PROGRAM MAIN
VAR
	master,slave:					axis_ref;
	camming_state: 					camming_state;
	
	camin:							mc_camin;(*用于电子凸轮耦合功能块*)
	camout:							mc_camout;(*用于电子凸轮表解耦功能块*)
	CamTableSelect_1:				MC_CamTableSelect;(*用于创建凸轮表*)
	cam_table1:						MC_CAM_REF;(*用于定义凸轮表*)
	table1: 						ARRAY[1..5] OF MC_MotionFunctionPoint; (*用于定义电子凸轮表中的关键点，此例子中包含五个关键点*)
	CamInOut,CamOutOut,selectOut:	ST_McOutputs;(*用于绑定相关功能块输出接口*)

	move_velo_master:				mc_movevelocity;
	move_abs_slave:					mc_moveabsolute;
	MoveMasterOut:					ST_McOutputs;		
	MoveSlaveOut:					ST_McOutputs;	

	ResetSlave,resetMaster:			mc_reset;	
	ResetMasterOut,ResetSlaveOut:	ST_McOutputs;
	
	master_actpos,slave_actpos:		LREAL;
END_VAR

(*用于更新轴状态*)
master();
slave();

power();
camming();
reset();
move_m_s();
table1_point();	

CASE camming_state OF
	state_init:(*程序初始化*)
		move_velo_master.Execute := FALSE;
		ResetMaster.Execute := FALSE;
		ResetSlave.Execute := FALSE;
		CamIn.Execute := FALSE;
		CamOut.Execute := FALSE;
		camming_state:=state_power;
	
	state_power:(*主从轴使能*)
		IF master.NcToPlc.StateDWord.0 AND master.NcToPlc.StateDWord.0 THEN
			camming_state := state_forward;
		ELSIF master.Status.Error OR slave.Status.Error THEN
			camming_state := state_error;
		END_IF	
	
	state_forward:(*主轴100正转，从轴回0*)
			move_velo_master.Execute:=TRUE;
			move_abs_slave. Execute:=TRUE;
			IF master.Status.Moving AND move_abs_slave.Done  THEN
				move_velo_master.Execute:=FALSE;
				move_abs_slave.Execute:=FALSE;
				camming_state:=state_pre_table1;
			END_IF
		IF master.Status.Error OR slave.Status.Error THEN
			camming_state := state_error;
		END_IF	
		
	state_pre_table1:(*table1初始化*)
		camtableselect_1.Execute:=TRUE;
		camin.CamTableID:=1;
		IF camtableselect_1.Done THEN
			camming_state:=state_camming1;
			camtableselect_1.Execute:=FALSE;
		END_IF
		IF master.Status.Error OR slave.Status.Error THEN
			camming_state := state_error;
		END_IF
	
	state_camming1:
		camin.Execute:=TRUE;
		IF camin.InSync THEN			
			camin.Execute:=FALSE;
			camming_state:=camming_status;		
		END_IF
		IF master.Status.Error OR slave.Status.Error THEN
			camming_state := state_error;
		END_IF
		
	camming_status:
		master_actpos:=master.NcToPlc.SetPos;
		slave_actpos:=slave.NcToPlc.SetPos;		
		IF master.Status.Error OR slave.Status.Error THEN
			camming_state := state_error;
		END_IF
		
	state_error:
		CamOut.Execute := Slave.Status.Coupled; (* 先解耦 *)		
		IF not Slave.Status.Coupled THEN
			IF Master.Status.Error OR Slave.Status.Error THEN
				camming_state := state_reset;	(* 轴报错需要reset*)
			ELSE
				camming_state  := state_init;(*若功能块报错，不需要reset*)
			END_IF
		END_IF
	
	state_reset:
		ResetMaster.Execute := TRUE;
		CamTableSelect_1.Execute:=FALSE;
			ResetSlave.Execute := TRUE;
			IF ResetMaster.Done AND ResetSlave.Done THEN
				camming_state := state_init;
			ELSIF ResetMaster.Error OR ResetSlave.Error THEN
				camming_state := state_init; 
			END_IF
	
END_CASE

ACTION camming:
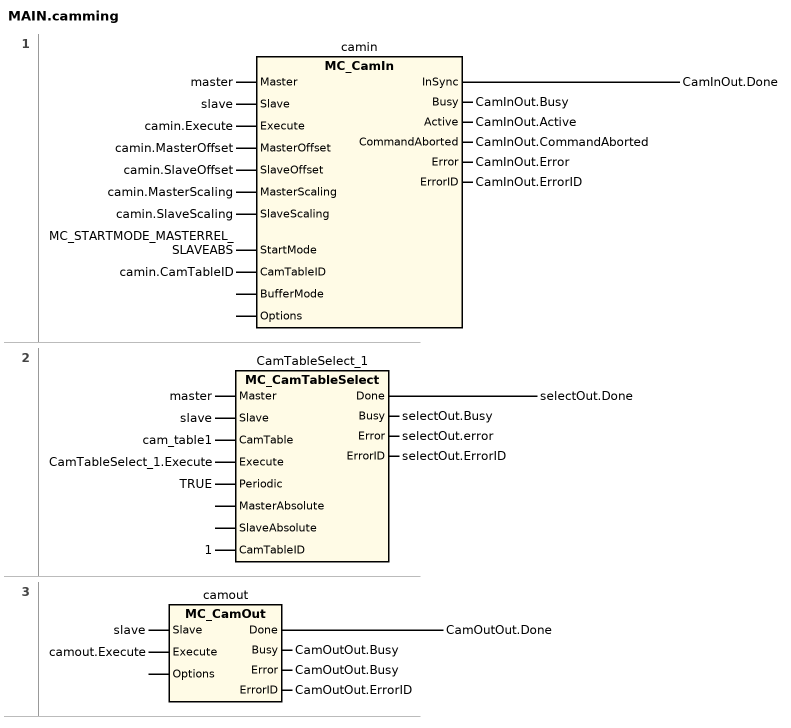
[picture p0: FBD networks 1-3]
// NETWORK 1
camin(
    Master := master,
    Slave := slave,
    Execute := camin.Execute,
    MasterOffset := camin.MasterOffset,
    SlaveOffset := camin.SlaveOffset,
    MasterScaling := camin.MasterScaling,
    SlaveScaling := camin.SlaveScaling,
    StartMode := MC_STARTMODE_MASTERREL_SLAVEABS,
    CamTableID := camin.CamTableID,
    Busy => CamInOut.Busy,
    Active => CamInOut.Active,
    CommandAborted => CamInOut.CommandAborted,
    Error => CamInOut.Error,
    ErrorID => CamInOut.ErrorID); // MC_CamIn
CamInOut.Done := camin.InSync;

// NETWORK 2
CamTableSelect_1(
    Master := master,
    Slave := slave,
    CamTable := cam_table1,
    Execute := CamTableSelect_1.Execute,
    Periodic := TRUE,
    CamTableID := 1,
    Busy => selectOut.Busy,
    Error => selectOut.error,
    ErrorID => selectOut.ErrorID); // MC_CamTableSelect
selectOut.Done := CamTableSelect_1.Done;

// NETWORK 3
camout(
    Slave := slave,
    Execute := camout.Execute,
    Busy => CamOutOut.Busy,
    Error => CamOutOut.Busy,
    ErrorID => CamOutOut.ErrorID); // MC_CamOut
CamOutOut.Done := camout.Done;
END_ACTION

ACTION move_m_s:
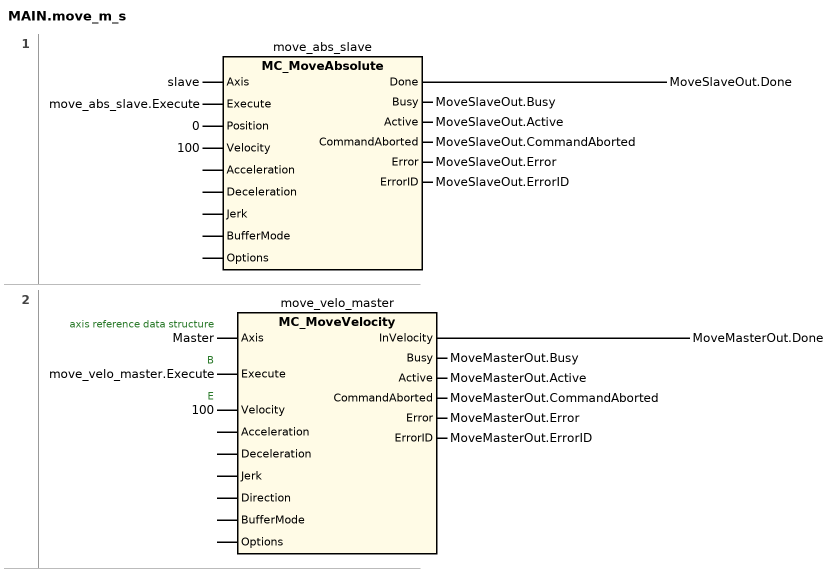
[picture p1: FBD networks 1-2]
// NETWORK 1
move_abs_slave(
    Axis := slave,
    Execute := move_abs_slave.Execute,
    Position := 0,
    Velocity := 100,
    Busy => MoveSlaveOut.Busy,
    Active => MoveSlaveOut.Active,
    CommandAborted => MoveSlaveOut.CommandAborted,
    Error => MoveSlaveOut.Error,
    ErrorID => MoveSlaveOut.ErrorID); // MC_MoveAbsolute
MoveSlaveOut.Done := move_abs_slave.Done;

// NETWORK 2
//   Master: axis reference data structure
//   move_velo_master.Execute: B
//   100: E
move_velo_master(
    Axis := Master,
    Execute := move_velo_master.Execute,
    Velocity := 100,
    Busy => MoveMasterOut.Busy,
    Active => MoveMasterOut.Active,
    CommandAborted => MoveMasterOut.CommandAborted,
    Error => MoveMasterOut.Error,
    ErrorID => MoveMasterOut.ErrorID); // MC_MoveVelocity
MoveMasterOut.Done := move_velo_master.InVelocity;
END_ACTION

ACTION power:
master.PlcToNc.ControlDWord:=7;
slave.PlcToNc.ControlDWord:=7;

master.PlcToNc.Override:=1000000;
slave.PlcToNc.Override:=1000000;
END_ACTION

ACTION reset:
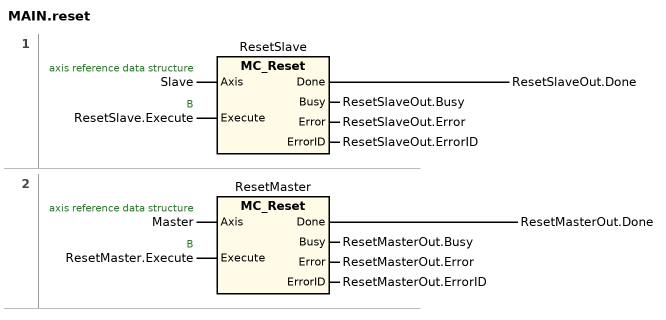
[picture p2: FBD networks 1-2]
// NETWORK 1
//   Slave: axis reference data structure
//   ResetSlave.Execute: B
ResetSlave(
    Axis := Slave,
    Execute := ResetSlave.Execute,
    Busy => ResetSlaveOut.Busy,
    Error => ResetSlaveOut.Error,
    ErrorID => ResetSlaveOut.ErrorID); // MC_Reset
ResetSlaveOut.Done := ResetSlave.Done;

// NETWORK 2
//   Master: axis reference data structure
//   ResetMaster.Execute: B
ResetMaster(
    Axis := Master,
    Execute := ResetMaster.Execute,
    Busy => ResetMasterOut.Busy,
    Error => ResetMasterOut.Error,
    ErrorID => ResetMasterOut.ErrorID); // MC_Reset
ResetMasterOut.Done := ResetMaster.Done;
END_ACTION

ACTION table1_point:
cam_table1.ArraySize:=SIZEOF(table1);
cam_table1.NoOfColumns:=1;
cam_table1.NoOfRows:=5;
cam_table1.pArray:=ADR(table1);
cam_table1.TableType:=MC_TABLETYPE_MOTIONFUNCTION;

		
table1[1].FunctionType:=MOTIONFUNCTYPE_POLYNOM5;
table1[1].MasterPos:=0;
table1[1].SlavePos:=0;
table1[1].PointIndex:=1;
table1[1].PointType:=MOTIONPOINTTYPE_MOTION;
		
table1[2].FunctionType:=MOTIONFUNCTYPE_POLYNOM5;
table1[2].MasterPos:=90;
table1[2].SlavePos:=100;
table1[2].PointIndex:=2;
table1[2].PointType:=MOTIONPOINTTYPE_MOTION;
		
table1[3].FunctionType:=MOTIONFUNCTYPE_POLYNOM5;
table1[3].MasterPos:=180;
table1[3].SlavePos:=80;
table1[3].PointIndex:=3;
table1[3].PointType:=MOTIONPOINTTYPE_MOTION;	
		
table1[4].FunctionType:=MOTIONFUNCTYPE_POLYNOM5;
table1[4].MasterPos:=270;
table1[4].SlavePos:=50;
table1[4].PointIndex:=4;
table1[4].PointType:=MOTIONPOINTTYPE_MOTION;
		
table1[5].FunctionType:=MOTIONFUNCTYPE_POLYNOM5;
table1[5].MasterPos:=360;
table1[5].SlavePos:=0;
table1[5].PointIndex:=5;
table1[5].PointType:=MOTIONPOINTTYPE_MOTION;
END_ACTION

END_PROGRAM
